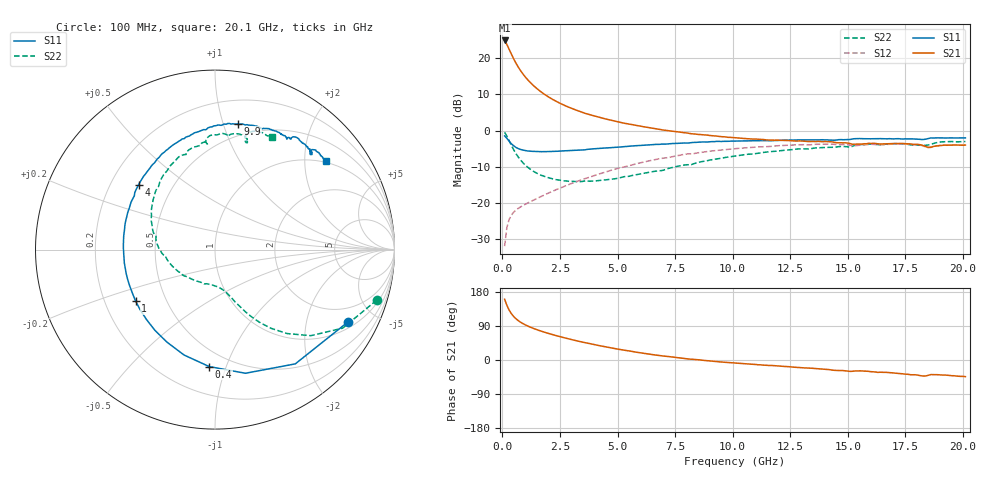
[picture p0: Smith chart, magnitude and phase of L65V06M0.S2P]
!  Infineon Technologies AG
! BFR380L3 , PF131585-7, No.6, Th 09.10.01, soldered on pcb-board, measured with PP GSG850
!  Vce=5.0 V,  Ic=6.0 mA
! Common Emitter S-Parameters:  15. November 2001
#  GHz  S  MA  R  50
! f  S11  S21  S12  S22
! GHz  Mag  Ang  Mag  Ang  Mag  Ang  Mag  Ang
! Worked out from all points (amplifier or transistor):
!   201 points, 100 MHz to 20.1 GHz, reference 50 ohm
!   highest |S21| = 25.0 dB at 100 MHz (marker M1)
!   |S21| within 3 dB of that: start of sweep to 335.7 MHz
!   unconditionally stable (mu >= 1): 2.17 GHz to 4.527 GHz
!   at 3.4 GHz: K = 1.04, MAG = 8.3 dB, |S12| = -13.7 dB
!   at 10.1 GHz: K = 0.93, MSG = 1.5 dB, |S12| = -5.0 dB
!   at 20.1 GHz: K = 0.99, MSG = 0.0 dB, |S12| = -4.0 dB
!   S11 on the Smith chart (normalised r, x): 100 MHz: 1.25, -3.48; 400 MHz: 0.39, -0.88; 1 GHz: 0.33, -0.27; 4 GHz: 0.32, +0.33; 9.9 GHz: 0.39, +1.12; 20.1 GHz: 0.96, +2.53
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0.1  0.8421 -28.8  17.73 160.4  0.02491 73.8  0.9442 -17.3
0.2  0.7782 -54.9  15.54 144.0  0.0455 63.2  0.8354 -31.6
0.3  0.7095 -76.2  13.28 131.4  0.05882 55.3  0.7177 -41.9
0.4  0.6526 -92.8  11.33 121.7  0.06763 49.9  0.6168 -49.3
0.5  0.612 -106.4  9.751 114.3  0.0741 47.2  0.537 -54.7
0.6  0.5808 -117.5  8.5 108.5  0.0793 45.4  0.4748 -58.5
0.7  0.5607 -126.6  7.512 103.6  0.08357 44.6  0.4258 -61.5
0.8  0.5455 -134.4  6.708 99.4  0.08764 44.4  0.3871 -63.9
1  0.5273 -147.0  5.521 92.7  0.09508 44.8  0.3313 -67.4
1.2  0.5168 -156.7  4.681 87.1  0.1025 45.9  0.2931 -70.3
1.4  0.5125 -164.9  4.066 82.2  0.1103 47.2  0.2662 -72.9
1.9  0.5103 179.6  3.071 72.0  0.1312 50.0  0.2269 -79.2
2.6  0.5213 163.7  2.306 60.1  0.1636 52.2  0.2029 -89.8
3.5  0.5395 147.2  1.772 46.9  0.211 52.3  0.1972 -105.1
4  0.5589 139.7  1.591 40.6  0.2381 51.5  0.1998 -115.9
5.3  0.5987 122.6  1.26 25.7  0.3127 46.6  0.2294 -142.3
6.8  0.6417 105.5  1.041 11.8  0.405 38.1  0.277 -171.3
9.9  0.7121 79.7  0.8037 -7.0  0.5524 17.1  0.4326 143.6
10.1  0.7139 78.4  0.7938 -8.2  0.5595 15.8  0.4429 141.1
13.5  0.7421 60.0  0.7052 -22.1  0.6395 -7.0  0.5674 105.9
16.8  0.771 47.9  0.6572 -33.2  0.6437 -24.1  0.6531 81.1
20.1  0.7903 38.6  0.6287 -43.9  0.6326 -38.2  0.7042 63.4
